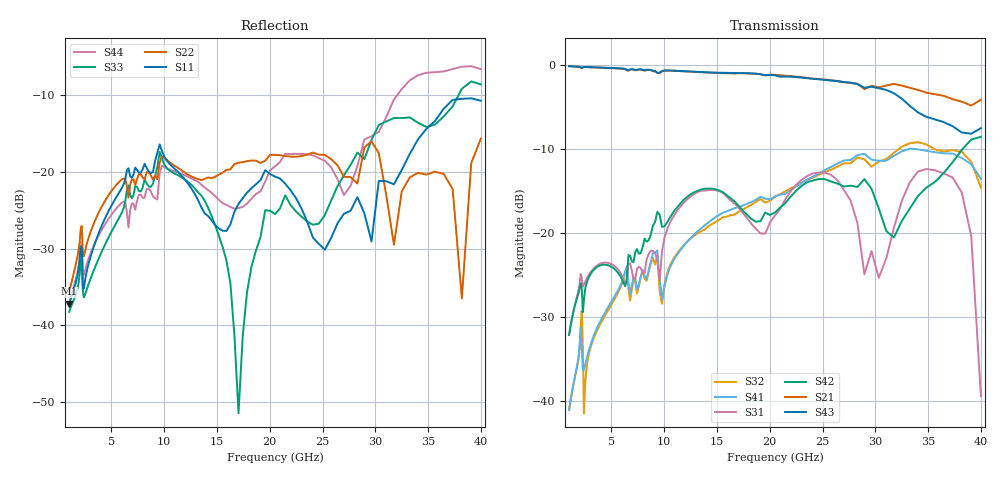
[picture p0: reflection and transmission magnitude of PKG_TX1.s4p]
! Created Mon Sep 18 16:11:09 2017
# hz S ma R 50
! 4 Port Network Data from SP1.SP block
! freq  magS11  angS11  magS12  angS12  magS13  angS13  magS14  angS14
!  magS21  angS21  magS22  angS22  magS23  angS23  magS24  angS24
!  magS31  angS31  magS32  angS32  magS33  angS33  magS34  angS34
!  magS41  angS41  magS42  angS42  magS43  angS43  magS44  angS44
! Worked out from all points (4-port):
!   161 points, 1 GHz to 40 GHz, reference 50 ohm
!   strongest paths, dB at 1 GHz, 2.515 GHz, 6.325 GHz, 15.91 GHz, 40 GHz:
!     S43: -0.1, -0.2, -0.4, -0.9, -7.5
!     S21: -0.1, -0.2, -0.5, -0.9, -4.1
!     S42: -32.2, -26.7, -26.3, -15.5, -8.5
!     S31: -32.1, -25.8, -26.2, -15.6, -39.4
!     S41: -41.1, -35.7, -24.5, -17.4, -13.5
!     S32: -41.1, -38.2, -24.7, -18.1, -14.6
!   lowest |S11| = -37.2 dB at 1 GHz (marker M1), VSWR 1.03, Z = 50.9 + j1.11 ohm
!   |S11| at or under -10 dB: start of sweep to end of sweep
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1e9  0.01384 51.7  0.9878 -18.8  0.02472 66.6  0.008856 -113.2
     0.9878 -18.8  0.01644 26.6  0.008818 -113.4  0.02465 72.9
     0.02472 66.6  0.008818 -113.4  0.01223 44.2  0.9882 -18.1
     0.008856 -113.2  0.02465 72.9  0.9882 -18.1  0.01387 26.1
1.002969e10  0.1253 -62.1  0.9291 177.9  0.09364 146.3  0.04814 89.7
             0.9291 177.9  0.1234 -118.6  0.04908 102.6  0.1096 34.9
             0.09364 146.3  0.04908 102.6  0.1113 -64.0  0.9313 -176.0
             0.04814 89.7  0.1096 34.9  0.9313 -176.0  0.1078 -105.3
1.704447e10  0.06188 50.1  0.896 49.4  0.1423 -40.4  0.1428 -43.1
             0.896 49.4  0.1149 -131.1  0.1337 -29.5  0.1453 -25.2
             0.1423 -40.4  0.1337 -29.5  0.002665 87.1  0.8995 59.3
             0.1428 -43.1  0.1453 -25.2  0.8995 59.3  0.05822 -127.3
2.464845e10  0.03399 -95.7  0.8281 -92.0  0.2296 60.4  0.2262 174.2
             0.8281 -92.0  0.1298 -157.2  0.2223 -170.6  0.2101 -55.0
             0.2296 60.4  0.2223 -170.6  0.046 -70.0  0.8251 -78.8
             0.2262 174.2  0.2101 -55.0  0.8251 -78.8  0.1232 -153.6
3.326266e10  0.1313 72.9  0.7348 107.1  0.2002 90.1  0.3185 -11.7
             0.7348 107.1  0.09224 -144.3  0.3431 12.2  0.1399 160.2
             0.2002 90.1  0.3431 12.2  0.2271 161.5  0.5739 115.4
             0.3185 -11.7  0.1399 160.2  0.5739 115.4  0.3965 173.2
3.819744e10  0.3003 -48.3  0.6066 15.4  0.1739 -20.4  0.2798 -128.2
             0.6066 15.4  0.01496 61.8  0.3045 -106.6  0.3135 81.2
             0.1739 -20.4  0.3045 -106.6  0.3494 -25.1  0.3973 43.6
             0.2798 -128.2  0.3135 81.2  0.3973 43.6  0.4864 74.4
4e10  0.2917 -80.0  0.6235 -11.5  0.01067 17.1  0.2106 -165.4
      0.6235 -11.5  0.1652 -109.3  0.1864 -151.3  0.3746 49.5
      0.01067 17.1  0.1864 -151.3  0.3729 -79.2  0.4219 22.2
      0.2106 -165.4  0.3746 49.5  0.4219 22.2  0.4693 37.8
